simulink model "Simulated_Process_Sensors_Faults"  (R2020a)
settings: Solver=ode45  StartTime=0  StopTime=300  MaxStep=0.02  RelTol=1e-3  AbsTol=1e-6
PreLoadFcn:
  | init_params_FS
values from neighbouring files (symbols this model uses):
  g = 9.8    [init_params_FS.m]
  K = [-3.1623 -4.8648 -45.9014 -14.6871]    [init_params_FS.m]
  l = 1    [init_params_FS.m]
  m = 0.1    [init_params_FS.m]
  M = 1    [init_params_FS.m]
  theta0 = 0.55    [init_params_FS.m]
  Ts = 0.05    [init_params_FS.m]
  x0 = 0.2    [init_params_FS.m]

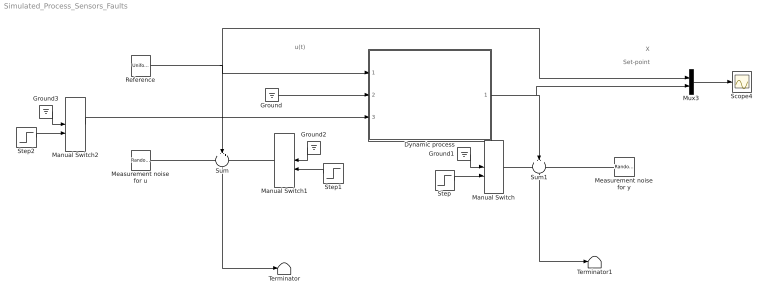
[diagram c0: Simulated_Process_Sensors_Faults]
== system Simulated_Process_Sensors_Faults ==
  note: u(t)
  note: Set-point
  note: X
  Dynamic process : Subsystem
  Ground{,1..3} (4 alike) : Ground
  Manual Switch : ManualSwitch
  Manual Switch1 : ManualSwitch
  Manual Switch2 : ManualSwitch
  Measurement noise for u : RandomNumber  Variance=0.00001  Seed=7  SampleTime=Ts
  Measurement noise for y : RandomNumber  Variance=0.000001  Seed=6  SampleTime=Ts
  Mux3 : Mux  Inputs=2
  Reference : UniformRandomNumber  Minimum=-0.3  Maximum=0.3  Seed=2  SampleTime=10
  Scope4 : Scope
  Step : Step  Time=150  SampleTime=0
  Step1 : Step  Time=150  SampleTime=0
  Step2 : Step  Time=150  After=2.1  SampleTime=0
  Sum : Sum  Inputs=+++
  Sum1 : Sum  Inputs=+++
  Terminator : Terminator
  Terminator1 : Terminator
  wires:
  Reference/1 -> Sum/2, Dynamic process/1(u1), Mux3/1
  Mux3/1 -> Scope4/1
  Dynamic process/1(y) -> Sum1/2, Mux3/2
  Measurement noise for u/1 -> Sum/1
  ? -> ?
  Measurement noise for y/1 -> Sum1/3
  Manual Switch1/1 -> Sum/3
  Sum1/1 -> Terminator1/1
  Step/1 -> Manual Switch/2
  Manual Switch/1 -> Sum1/1
  Ground1/1 -> Manual Switch/1
  Ground2/1 -> Manual Switch1/1
  Step1/1 -> Manual Switch1/2
  Ground/1 -> Dynamic process/2(u2)
  Manual Switch2/1 -> Dynamic process/3(fs)
  Step2/1 -> Manual Switch2/2
  Ground3/1 -> Manual Switch2/1
  Sum/1 -> Terminator/1

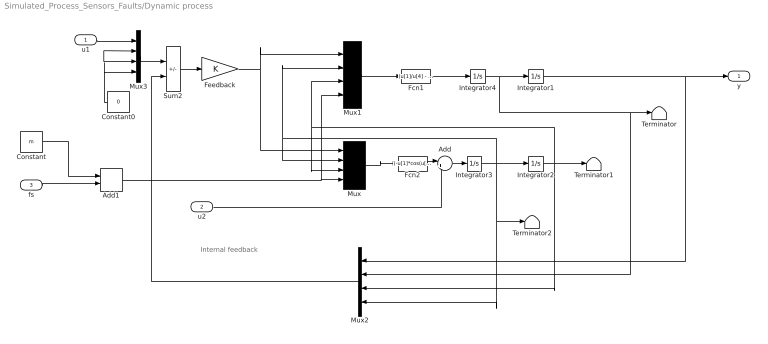
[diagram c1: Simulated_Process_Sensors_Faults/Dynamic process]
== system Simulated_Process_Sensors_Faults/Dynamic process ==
  note: Internal feedback
  u1 : Inport
  u2 : Inport  Port=2
  fs : Inport  Port=3
  Add : Sum  Inputs=|++  InputSameDT=on
  Add1 : Sum
  Constant : Constant  Value=m
  Constant0 : Constant  Value=0
  Fcn1 : Fcn  Expr=(u[1]/u[4] - g*sin(u[3])*cos(u[3]) + l*power(u[2],2)*sin(u[3]))/(M/u[4] + power(sin(u[3]),2))
  Fcn2 : Fcn  Expr=(-u[1]*cos(u[3])/u[4] + (M+u[4])*g*sin(u[3])/u[4] - l*power(u[2],2)*sin(u[3])*cos(u[3]))/(l*(M/u[4] + power(sin(u[3]),2)))
  Feedback : Gain  Gain=K  Multiplication=Matrix(K*u)
  Integrator1 : Integrator  InitialCondition=x0
  Integrator2 : Integrator  InitialCondition=theta0
  Integrator3 : Integrator
  Integrator4 : Integrator
  Mux{,1..3} (4 alike) : Mux
  Sum2 : Sum  Inputs=+-  InputSameDT=on  SaturateOnIntegerOverflow=on
  Terminator : Terminator
  Terminator1 : Terminator
  Terminator2 : Terminator
  y : Outport
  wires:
  Mux/1 -> Fcn2/1
  Mux1/1 -> Fcn1/1
  Fcn1/1 -> Integrator4/1
  Integrator4/1 -> Integrator1/1, Mux2/2, Terminator/1
  Feedback/1 -> Mux/1, Mux1/1
  Integrator3/1 -> Mux1/2, Mux/2, Integrator2/1, Mux2/4, Terminator2/1
  Integrator2/1 -> Mux1/3, Mux/3, Mux2/3, Terminator1/1
  Add/1 -> Integrator3/1
  Fcn2/1 -> Add/1
  Integrator1/1 -> y/1, Mux2/1
  u2/1 -> Add/2
  Sum2/1 -> Feedback/1
  Constant0/1 -> Mux3/2, Mux3/3, Mux3/4
  Mux3/1 -> Sum2/1
  u1/1 -> Mux3/1
  Mux2/1 -> Sum2/2
  Add1/1 -> Mux1/4, Mux/4
  Constant/1 -> Add1/1
  fs/1 -> Add1/2
